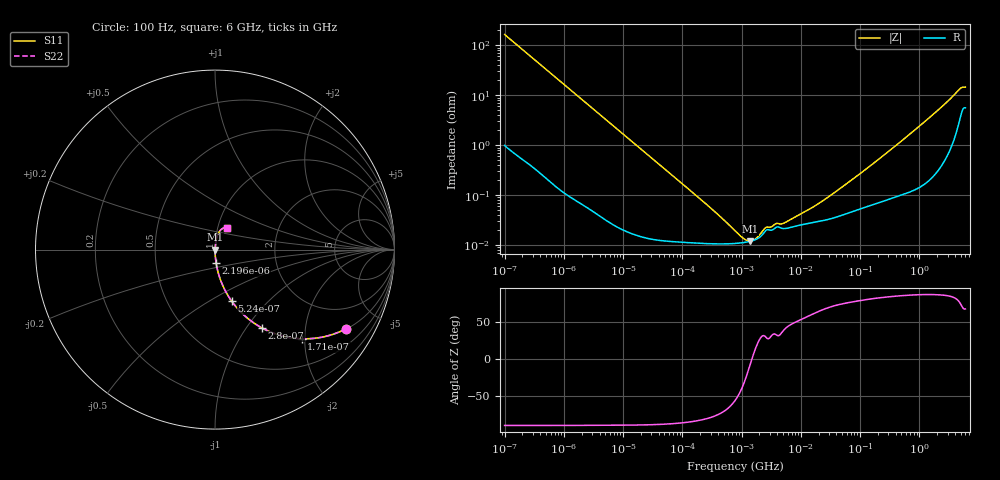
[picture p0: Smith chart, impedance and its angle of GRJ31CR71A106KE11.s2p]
!Murata Part Number: GRJ31CR71A106KE11
!These Parameters are Measured in Series Mode Connection
!Data Generated on Jun 19, 2026
!  o--ll--o
!Port1  Port2
!  o------o
!Operation Temp=25[degC], DC Bias Voltage=0[V]
!Freq. Start=100[Hz] Stop=6[GHz] 401[Steps]
# Hz S RI R 50
!Freq.(Hz) S11(Real) S11(Imag) S21(Real) S21(Imag) S12(Real) S12(Imag) S22(Real) S22(Imag)
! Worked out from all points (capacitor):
!   401 points, 100 Hz to 6 GHz, reference 50 ohm
!   read as one part in series: C = 9.63 uF near 109 Hz
!   lowest |Z| = 12.1 mohm at 1.386 MHz (marker M1)
!   series resonance near 1.496 MHz, so ESL is about 1.2 nH
!   S11 on the Smith chart (normalised r, x): 100 Hz: 1.02, -3.30; 171 Hz: 1.01, -1.93; 280 Hz: 1.01, -1.18; 524 Hz: 1.00, -0.63; 2.196 kHz: 1.00, -0.15; 6 GHz: 1.11, +0.27
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100  0.7303 -0.4408  0.2697 0.4408  0.2697 0.4408  0.7303 -0.4408
171  0.4829 -0.4966  0.5171 0.4966  0.5171 0.4966  0.4829 -0.4966
280  0.2606 -0.4357  0.7394 0.4357  0.7394 0.4357  0.2606 -0.4357
524  0.0928 -0.2869  0.9072 0.2869  0.9072 0.2869  0.0928 -0.2869
981  0.029 -0.1646  0.971 0.1646  0.971 0.1646  0.029 -0.1646
2008  0.00751 -0.0825  0.9925 0.0825  0.9925 0.0825  0.00751 -0.0825
2196  0.00635 -0.0755  0.9936 0.0755  0.9936 0.0755  0.00635 -0.0755
6728  0.000879 -0.0249  0.9991 0.0249  0.9991 0.0249  0.000879 -0.0249
40335  0.000142 -0.00418  0.9999 0.00418  0.9999 0.00418  0.000142 -0.00418
289253  0.000107 -0.000567  0.9999 0.000567  0.9999 0.000567  0.000107 -0.000567
774597  0.000108 -0.000162  0.9999 0.000162  0.9999 0.000162  0.000108 -0.000162
1108252  0.000113 -6.99e-05  0.9999 6.99e-05  0.9999 6.99e-05  0.000113 -6.99e-05
1386327  0.000119 -1.76e-05  0.9999 1.76e-05  0.9999 1.76e-05  0.000119 -1.76e-05
1734173  0.00013 3.47e-05  0.9999 -3.47e-05  0.9999 -3.47e-05  0.00013 3.47e-05
2594782  0.000199 0.000111  0.9998 -0.000111  0.9998 -0.000111  0.000199 0.000111
5311619  0.000215 0.00018  0.9998 -0.00018  0.9998 -0.00018  0.000215 0.00018
1.555665e7  0.000282 0.00049  0.9997 -0.00049  0.9997 -0.00049  0.000282 0.00049
5.211241e7  0.000407 0.00146  0.9996 -0.00146  0.9996 -0.00146  0.000407 0.00146
3.124326e8  0.000892 0.0077  0.9991 -0.0077  0.9991 -0.0077  0.000892 0.0077
1.637704e9  0.00378 0.0393  0.9962 -0.0393  0.9962 -0.0393  0.00378 0.0393
4.586474e9  0.0391 0.1159  0.9609 -0.1159  0.9609 -0.1159  0.0391 0.1159
6e9  0.0683 0.1187  0.9317 -0.1187  0.9317 -0.1187  0.0683 0.1187
